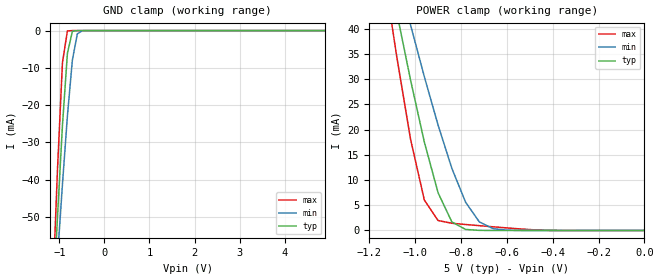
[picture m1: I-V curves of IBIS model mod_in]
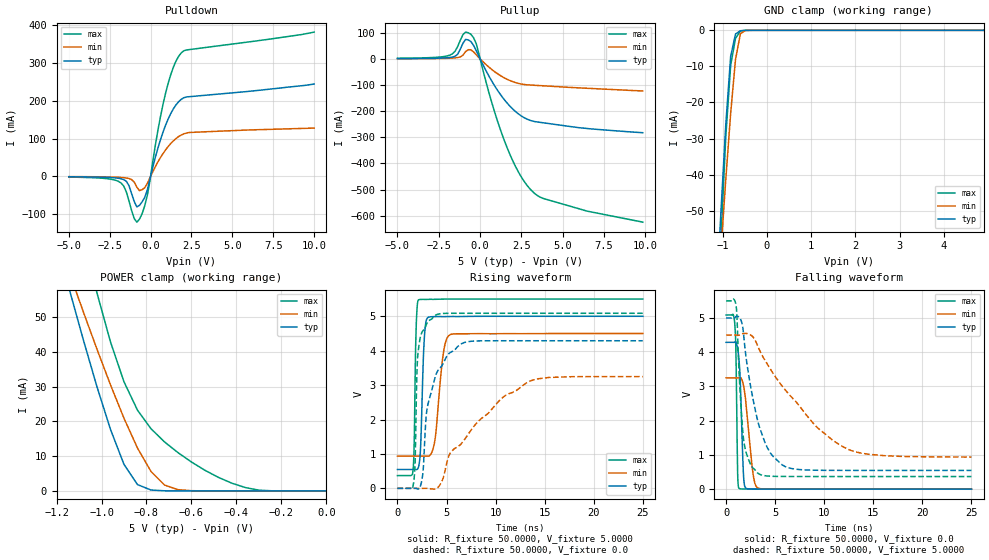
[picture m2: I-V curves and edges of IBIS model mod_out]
| IBIS (I/O, Buffer, Information, Specification) Model, officially
| electronic behavioral standard for Buffer structures of digital pins.
[IBIS ver]  4.0
[File name] 54act240_5v0_rev1.ibs
[File Rev]  1.0
[Date]   24 Nov 2016
[Source]   CAD & Design Services (Catania) - STMicroelectronics
[Notes]
  (Note1) This IBIS model is the model of the product with package
   (Flat20 package elements);
  (Note2) This IBIS model is extracted with nominal 5.0V power supply
   (min:4.5V, typ:5.0V, max:5.5V);
  (Note3) This model has few Warnings about the non-monotonicity
   of I-V curves, but they are not indicative of problems
   inside the model;
[Copyright] (c) 2016 STMicroelectronics
|   Component RHFACT240
[Component] RHFACT240
[Manufacturer] STMicroelectronics
[Package]
| variable  typ   min   max
R_pkg   0.0   0.0   0.0
L_pkg   0.0H   0.0H   0.0H
C_pkg   0.0F   0.0F   0.0F
[Pin]   signal_name   model_name   R_pin   L_pin   C_pin
1   OE1   mod_in   178.9m   6.2nH   1.2pF
2   1A1   mod_in   182.5m   6.3nH   1.2pF
3   4Y2   mod_out   114.4m   3.5nH   1.3pF
4   2A1   mod_in   79.1m   2.3nH   0.9pF
5   3Y2   mod_out   75.8m   2.2nH   0.8pF
6   3A1   mod_in   75.8m   2.2nH   0.8pF
7   2Y2   mod_out   84.5m   2.4nH   0.9pF
8   4A1   mod_in   116.2m   3.6nH   1.3pF
9   1Y2   mod_out   178.9m   6.2nH   1.2pF
10   GND   GND   117.4m   4.4nH   1.2pF
11   1A2   mod_in   178.9m   6.2nH   1.2pF
12   4Y1   mod_out   189.6m   6.6nH   1.2pF
13   2A2   mod_in   125.1m   3.9nH   1.3pF
14   3Y1   mod_out   86.3m   2.5nH   0.9pF
15   3A2   mod_in   79.4m   2.3nH   0.8pF
16   2Y1   mod_out   75.8m   2.2nH   0.8pF
17   4A2   mod_in   75.6m   2.1nH   0.9pF
18   1Y1   mod_out   89.3m   2.7nH   1.3pF
19   OE2   mod_in   184.3m   6.4nH   1.2pF
20   VCC   POWER   118.0m   4.4nH   1.2pF
| Models and submodels in the file (2): mod_in (Input), mod_out (3-state)
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|   Model mod_in
[Model]   mod_in
Model_type Input
Vinl   =   0.8000V
Vinh   =   2.0000V
C_comp   0.532pF   0.386pF   0.702pF
[Temperature Range]  25.0000   0.1250k   -55.0000
[Voltage Range]   5.0000V   4.5000V   5.5000V
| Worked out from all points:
|   GND clamp passes 1 mA (typ) near -0.72 V on its own axis
|   POWER clamp passes 1 mA (typ) near -0.81 V on its own axis
[GND_clamp]
|Voltage   I(typ)   I(min)   I(max)
-5V       -1.077A    -851mA     -1.388A
-1.15V    -76.21mA   -81.38mA   -71.15mA
-1.04V    -49.97mA   -60.95mA   -37.22mA
-930mV    -25.45mA   -41.23mA   -8.617mA
-820mV    -6.089mA   -22.9mA    -92.5uA
-710mV    -201.6uA   -7.912mA   -269.9nA
-600mV    -2.872uA   -880.8uA   -788.8pA
-490mV    -39.72nA   -40.32uA   -14.69pA
4.9V      9.601pA    192.6nA    9.1pA
[POWER_clamp]
|Voltage   I(typ)   I(min)   I(max)
-4.98V    1.054A     828.1mA    1.363A
-1.14V    57.11mA    62.23mA    52.27mA
-1.08V    43.14mA    51.32mA    34.33mA
-1.02V    29.78mA    40.7mA     18.05mA
-960mV    17.52mA    30.47mA    6.025mA
-900mV    7.461mA    20.87mA    1.97mA
-840mV    1.695mA    12.32mA    1.432mA
-780mV    204.9uA    5.595mA    1.184mA
-720mV    20.39uA    1.698mA    952.8uA
-660mV    1.979uA    357.7uA    726.2uA
-600mV    191.5nA    64.88uA    506.4uA
0V        10pA       55.35pA    11.5pA
|   Model mod_out
[Model]   mod_out
Model_type 3-state
Polarity   Inverting
Enable   Active-Low
|Vinl  =   0.8000V
|Vinh  =   2.0000V
Vmeas  =   2.500V
Cref   =   50pF
Rref   =   500
Vref   =   5.000V
C_comp   2.668pF   2.119pF   3.517pF
[Temperature Range]  25.0000   0.1250k   -55.0000
[Voltage Range]   5.0000V   4.5000V   5.5000V
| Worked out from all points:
|   slope of the pulldown table from 0 to 0.75 V, typ, clamps not added: 6.47 ohm
|   slope of the pullup table from 0 to 0.75 V, typ, clamps not added: 8.35 ohm
|   GND clamp passes 1 mA (typ) near -0.71 V on its own axis
|   POWER clamp passes 1 mA (typ) near -0.81 V on its own axis
|   rising waveform, R_fixture 50.0000, V_fixture 5.0000: 20-80 % time 298ps typ, 683ps min, 178ps max; typ from 0.548 V to 5 V
|   rising waveform, R_fixture 50.0000, V_fixture 0.0: 20-80 % time 1.46ns typ, 5.61ns min, 331ps max; typ from 0 V to 4.29 V
|   falling waveform, R_fixture 50.0000, V_fixture 0.0: 20-80 % time 305ps typ, 668ps min, 152ps max; typ from 4.29 V to 0 V
|   falling waveform, R_fixture 50.0000, V_fixture 5.0000: 20-80 % time 1.93ns typ, 6.01ns min, 633ps max; typ from 5 V to 0.548 V
[Pulldown]
|Voltage   I(typ)   I(min)   I(max)
-5V       -1.1mA     -660uA     -2.1mA
-1.8V     -6.45mA    -2.86mA    -17.7mA
-1.32V    -24.82mA   -5.73mA    -65.26mA
-1V       -66.48mA   -15.2mA    -111.6mA
-840mV    -80.83mA   -28.56mA   -121.3mA
-520mV    -67.65mA   -35.3mA    -99.35mA
-200mV    -36.1mA    -18.88mA   -50.51mA
440mV     73.46mA    37.6mA     120mA
1.08V     152.3mA    79.23mA    247.1mA
1.56V     189.5mA    100.3mA    305.6mA
1.88V     204mA      109.5mA    327mA
10V       244.3mA    127.7mA    381.8mA
[Pullup]
|Voltage   I(typ)   I(min)   I(max)
-5V       900uA      550uA      2.2mA
-1.84V    5.14mA     2.39mA     14.04mA
-1.36V    17.51mA    4.89mA     46.98mA
-1.04V    59.48mA    13.79mA    92.34mA
-560mV    66.32mA    34.71mA    94.14mA
-240mV    32.4mA     15.97mA    59.22mA
720mV     -86.67mA   -41.45mA   -170.4mA
1.52V     -160.5mA   -74.53mA   -321.6mA
2.32V     -210.6mA   -93.95mA   -432.9mA
3.12V     -237.1mA   -100.3mA   -504.2mA
6.48V     -266.3mA   -112.5mA   -582.2mA
9.84V     -282.4mA   -122.7mA   -624.4mA
[GND_clamp]
|Voltage   I(typ)   I(min)   I(max)
-5V       -1.077A    -851mA     -1.394A
-1.15V    -76.48mA   -81.43mA   -89.92mA
-1.04V    -50.34mA   -61.01mA   -57.79mA
-930mV    -26.04mA   -41.3mA    -29.44mA
-820mV    -7.201mA   -23mA      -9.708mA
-710mV    -1.007mA   -8.036mA   -2.192mA
-600mV    -110.4uA   -960.7uA   -202.4uA
-490mV    -9.509uA   -58.05uA   -7.201uA
-380mV    -722.1nA   -4.418uA   -257.7nA
4.9V      105.2pA    197nA      -9.7nA
[POWER_clamp]
|Voltage   I(typ)   I(min)   I(max)
-4.98V    1.054A     828.1mA    1.383A
-1.14V    57.2mA     62.23mA    89.55mA
-1.08V    43.24mA    51.32mA    72.64mA
-1.02V    29.9mA     40.7mA     56.86mA
-960mV    17.66mA    30.47mA    42.81mA
-900mV    7.62mA     20.87mA    31.36mA
-840mV    1.821mA    12.32mA    23.21mA
-780mV    258.2uA    5.595mA    17.88mA
-720mV    36.77uA    1.698mA    14.1mA
-540mV    379.1nA    11.39uA    5.929mA
-360mV    7.779nA    63.84nA    960.3uA
0V        111.1pA    0A         0A
[Ramp]
| variable   typ   min   max
dV/dt_r  2.5731/1.5793n   1.9487/5.5651n   3.0520/0.5161n
dV/dt_f  2.6711/1.9509n   2.1382/5.9661n   3.0781/0.7601n
R_load = 50.0000
[Rising Waveform]
R_fixture= 50.0000
V_fixture= 5.0000
V_fixture_min= 4.5000
V_fixture_max= 5.5000
|time   V(typ)   V(min)   V(max)
0s        547.7mV    936.9mV    369.7mV
1.575ns   547.7mV    936.9mV    497.3mV
1.675ns   547.8mV    936.9mV    953.6mV
1.925ns   546.1mV    936.9mV    4.847V
2.175ns   649.9mV    936.9mV    5.48V
2.375ns   1.302V     936.9mV    5.489V
2.75ns    4.423V     936.9mV    5.49V
3.1ns     4.964V     935.2mV    5.491V
5.4ns     4.993V     4.47V      5.5V
25ns      5V         4.5V       5.5V
[Rising Waveform]
R_fixture= 50.0000
V_fixture= 0.0
V_fixture_min= 0.0
V_fixture_max= 0.0
|time   V(typ)   V(min)   V(max)
0s        145.2pV    260pV      62.5nV
1.575ns   -8.625uV   -1.016uV   47.72mV
1.8ns     337uV      -1.022uV   753.7mV
1.95ns    -4.45mV    -1.272uV   3.014V
2.125ns   -22.79mV   -1.963uV   4.014V
3ns       2.285V     699.5uV    4.796V
3.825ns   3.212V     -24.31mV   5.021V
6.8ns     4.237V     1.403V     5.087V
13.1ns    4.288V     3.057V     5.087V
25ns      4.288V     3.248V     5.087V
[Falling Waveform]
R_fixture= 50.0000
V_fixture= 0.0
V_fixture_min= 0.0
V_fixture_max= 0.0
|time   V(typ)   V(min)   V(max)
0s        4.288V     3.248V     5.087V
875ps     4.294V     3.248V     4.859V
975ps     4.303V     3.248V     4.314V
1.175ns   4.113V     3.247V     457.6mV
1.3ns     3.81V      3.249V     27.05mV
1.75ns    520.4mV    3.056V     5.289mV
1.975ns   32.65mV    2.638V     3.978mV
2.75ns    4.746mV    432.6mV    3.057mV
3.3ns     3.125mV    26.31mV    3.006mV
25ns      -402nV     13.88uV    -639.1nV
[Falling Waveform]
R_fixture= 50.0000
V_fixture= 5.0000
V_fixture_min= 4.5000
V_fixture_max= 5.5000
|time   V(typ)   V(min)   V(max)
0s        5V         4.5V       5.5V
1ns       5.043V     4.5V       5.385V
1.1ns     5.05V      4.5V       5.088V
1.4ns     4.997V     4.505V     2.976V
1.8ns     4.462V     4.544V     1.413V
3.3ns     1.905V     4.127V     452.7mV
4.5ns     1.061V     3.512V     378.5mV
6ns       661.2mV    2.907V     370.5mV
12.3ns    548mV      1.181V     369.7mV
25ns      547.7mV    937.9mV    369.7mV
